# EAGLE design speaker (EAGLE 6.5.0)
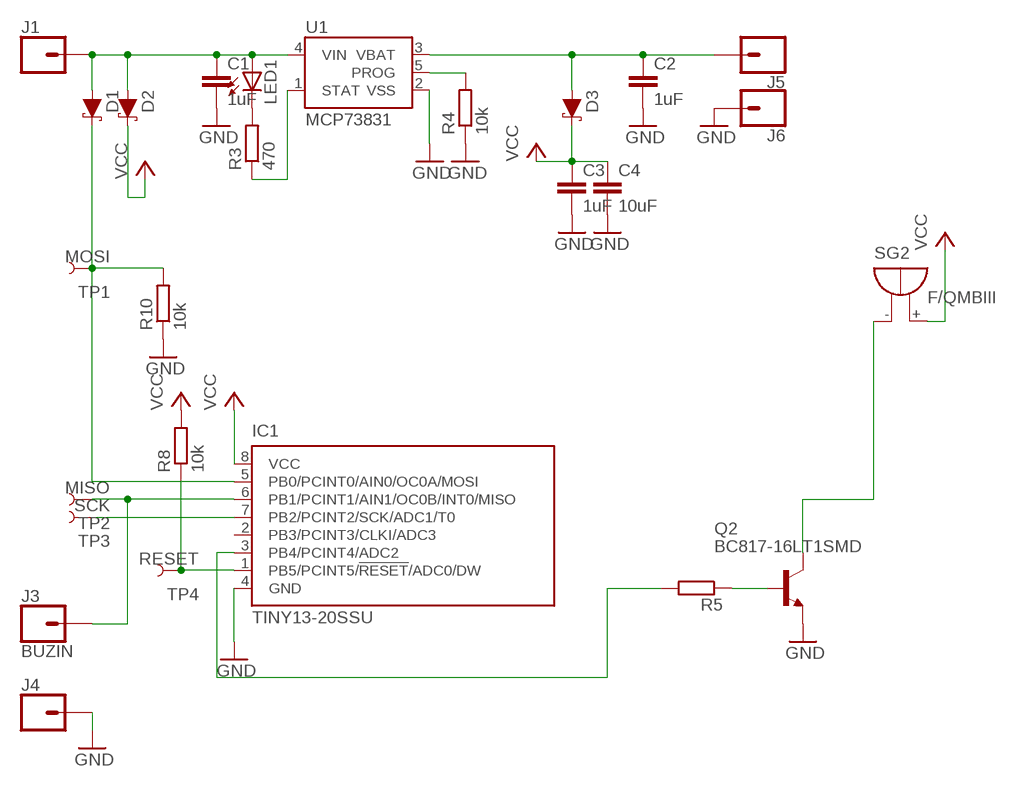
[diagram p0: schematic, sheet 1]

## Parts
C1  1uF  C-EUC1206  [C1206]
C2  1uF  C-EUC1206  [C1206]
C3  1uF  C-EUC1206  [C1206]
C4  10uF  C-EUC1206  [C1206]
D1  DIODE-SCHOTTKY-B340A  [SMA-DIODE]
D2  DIODE-SCHOTTKY-B340A  [SMA-DIODE]
D3  DIODE-SCHOTTKY-B340A  [SMA-DIODE]
IC1  TINY13-20SSU  [8S1]
J1  CONN_01OFFSET  [1X01_OFFSET]
J3  BUZIN  CONN_01OFFSET  [1X01_OFFSET]
J4  CONN_01OFFSET  [1X01_OFFSET]
J5  CONN_01OFFSET  [1X01_OFFSET]
J6  CONN_01OFFSET  [1X01_OFFSET]
LED1  LEDCHIP-LED0805  [CHIP-LED0805]
Q2  BC817-16LT1SMD  [SOT23-BEC]
R3  470  R-EU_M0805  [M0805]
R4  10k  R-EU_M0805  [M0805]
R5  R-EU_M0805  [M0805]
R8  10k  R-EU_M0805  [M0805]
R10  10k  R-EU_M0805  [M0805]
SG2  F/QMBIII  [F/QMBIII]
TP1  MOSI  TEST-POINT3X5  [PAD.03X.05]
TP2  MISO  TEST-POINT3X5  [PAD.03X.05]
TP3  SCK  TEST-POINT3X5  [PAD.03X.05]
TP4  RESET  TEST-POINT3X5  [PAD.03X.05]
U1  MCP73831  [SOT23-5]

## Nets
BUZER: Q2.C SG2.-(+)
GND: C1.2 C2.2 C3.2 C4.2 IC1.4(GND) J4.1 J6.1 Q2.E R4.1 R10.1 U1.2(VSS)
N$3: C1.1 D1.A D2.A J1.1 LED1.A U1.4(VIN)
N$4: LED1.C R3.2
N$6: R3.1 U1.1(STAT)
N$7: R4.2 U1.5(PROG)
N$8: C2.1 D3.A J5.1 U1.3(VBAT)
N$9: IC1.6(PB1/PCINT1/AIN1/OC0B/INT0/MISO) J3.1 TP2.P$1
N$10: IC1.1(PB5/PCINT5/!RESET!/ADC0/DW) R8.1 TP4.P$1
N$12: D1.C IC1.5(PB0/PCINT0/AIN0/OC0A/MOSI) R10.2 TP1.P$1
N$13: IC1.7(PB2/PCINT2/SCK/ADC1/T0) TP3.P$1
N$18: Q2.B R5.1
N$20: IC1.3(PB4/PCINT4/ADC2) R5.2
VCC: C3.1 C4.1 D2.C D3.C IC1.8(VCC) R8.2 SG2.+(-)
Unconnected: IC1.2(PB3/PCINT3/CLKI/ADC3)

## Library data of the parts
C1-C4 = rcl:C-EU: CAPACITOR, European symbol
D1-D3 = SparkFun-DiscreteSemi:DIODE-SCHOTTKY: Schottky diode; PROD_ID: DIO-09886; VALUE: 3A/40V/500mV
IC1 = atmel:TINY13: 8-bit AVR Microcontroller with 1K Bytes In-System Programmable Flash Source: http://www.atmel.com/dyn/resources/prod_documents/2535S.pdf; MPN: ATTINY13-20SSU; OC_FARNELL: 1455133; OC_NEWARK: 58M3771
J1 J3-J6 = SparkFun-Connectors:CONN_01: Single connection point. Often used as Generic Header-pin footprint for 0.1 inch spaced/style header connections
LED1 = led:LED: LED
Q2 = transistor-npn:BC817*: NPN Transistor
R3-R5 R8 R10 = rcl:R-EU_: RESISTOR, European symbol
SG2 = buzzer:F/QMBIII: BUZZER; OC_FARNELL: unknown; OC_NEWARK: unknown
TP1-TP4 = SparkFun-Connectors:TEST-POINT: SparkFun Test Points
U1 = SparkFun-IC-Power:MCP73831: MCP73831T Li-Ion, Li-Pol Controller Miniature single cell, fully integrated Li-Ion, Li-polymer charge management controller Datasheet SparkFun Products: SparkFun ESP32 Thing SparkFun 9DoF Razor IMU M0; PROD_ID: IC-09995

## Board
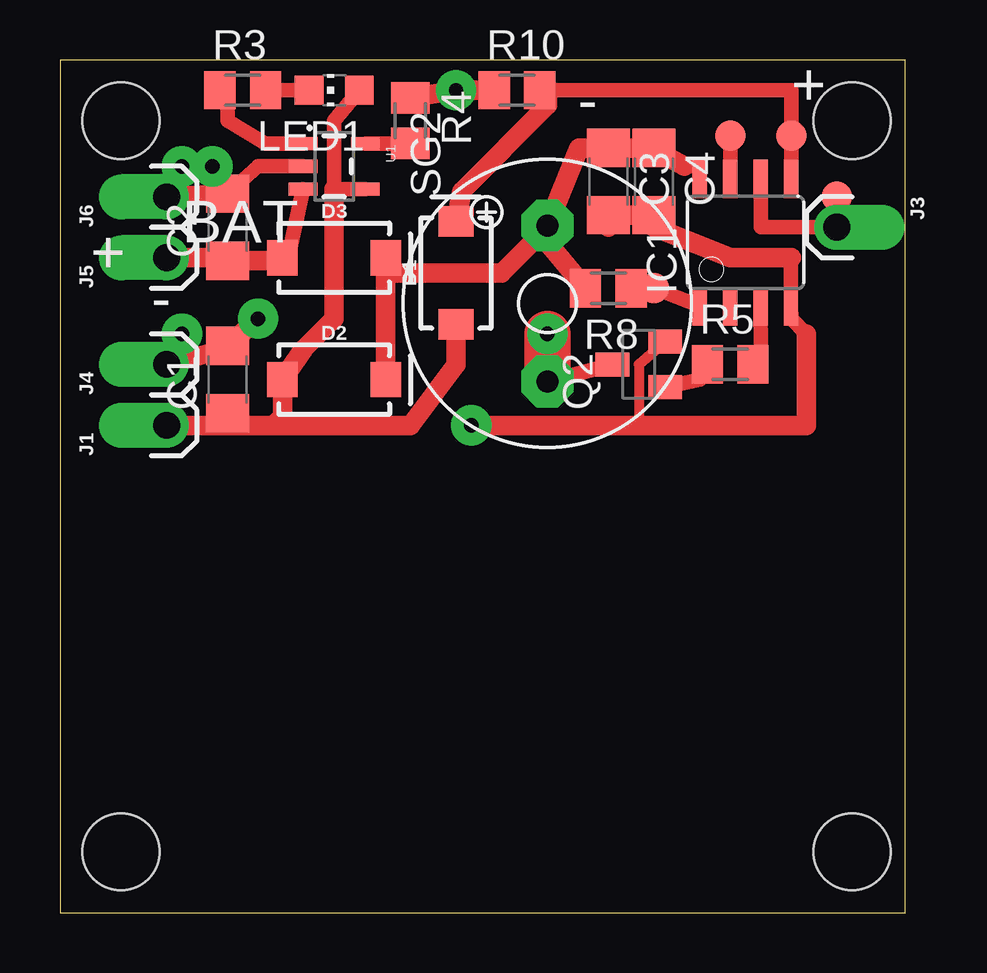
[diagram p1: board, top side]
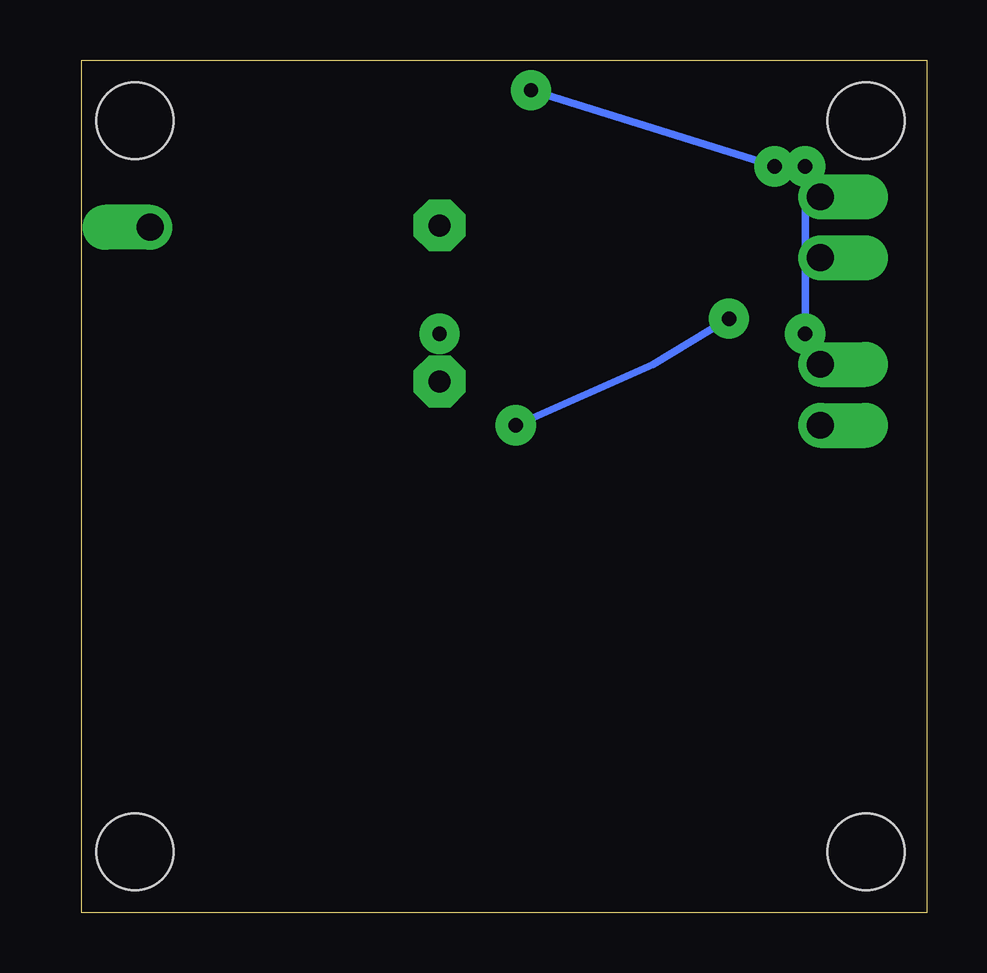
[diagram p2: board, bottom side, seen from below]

Size 35.23 x 35.55 mm. Coordinates in mm from the lower left corner, seen from the top.
Outline: 0,0 35.23,0 35.23,35.55 0,35.55 0,0
Copper layers (1*16): Top 0.035mm / dielectric 1.5mm / Bottom 0.035mm
Design rules "default": minimum track width 10mil, minimum drill 24mil, track to track 8mil, track to pad 8mil, pad to pad 8mil, via to via 8mil, smd to smd 8mil, copper to edge 40mil, drill to drill 8mil, minimum pad ring 10mil, minimum via ring 8mil, stop-mask expansion 4mil, vias tented up to drill 0mil, thermal gap 10mil
Holes 3.2 mm at 2.54,2.54 33.02,2.54 33.02,33.02 2.54,33.02

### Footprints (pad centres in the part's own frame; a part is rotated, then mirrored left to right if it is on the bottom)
C1206 = smd 1.6 x 1.8: 1 -1.4,0; 2 1.4,0
SMA-DIODE = smd 1.27 x 1.47: A -2.15,0; C 2.15,0
8S1 = smd 0.6 x 1.6: 1 -1.905,-2.654; 2 -0.645,-2.654; 3 0.625,-2.654; 4 1.895,-2.654; 5 1.905,2.654; 6 0.635,2.654; 7 -0.635,2.654; 8 -1.905,2.654
1X01_OFFSET = drill 1.118 pad 1.88 offset: 1 0,0
CHIP-LED0805 = smd 1.2 x 1.2: A 0,-1.05; C 0,1.05
SOT23-BEC = smd 1 x 1.4: B -0.95,-1.1; C 0,1.1; E 0.95,-1.1
M0805 = smd 1.3 x 1.6: 1 -0.95,0; 2 0.95,0
F/QMBIII = drill 0.914 pad 2.159 octagon: + 3.251,0; - -3.251,0
PAD.03X.05 = smd 1.27 x 1.27: P$1 0,0
SOT23-5 = smd 0.55 x 1.2: 1 -0.95,-1.3; 2 0,-1.3; 3 0.95,-1.3; 4 0.95,1.3; 5 -0.95,1.3

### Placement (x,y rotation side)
C1  6.99,22.23 90 top
C2  6.99,28.57 90 top
C3  22.86,30.48 270 top
C4  24.77,30.48 270 top
D1  16.51,26.67 90 top
D2  11.43,22.23 0 top
D3  11.43,27.3 0 top
IC1  28.57,27.94 0 top
J1  4.45,20.32 90 top
J3  32.38,28.57 270 top
J4  4.45,22.86 90 top
J5  4.45,27.3 90 top
J6  4.45,29.84 90 top
LED1  11.43,34.29 90 top
Q2  24.13,22.86 90 top
R3  7.62,34.29 0 top
R4  14.61,33.02 270 top
R5  27.94,22.86 0 top
R8  22.86,26.04 180 top
R10  19.05,34.29 0 top
SG2  20.32,25.4 90 top
TP1  30.48,32.38 0 top
TP2  32.38,29.84 0 top
TP3  27.94,32.38 0 top
TP4  24.77,26.04 0 top
U1  11.43,31.11 270 top

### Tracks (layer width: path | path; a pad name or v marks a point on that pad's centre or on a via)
BUZER
  Top 0.61: Q2.C SG2.-
GND  (via drill 0.6 pad 1.68)
  Top 0.406: Q2.E 24.13,22.86 24.13,20.32
  Top 0.61: U1.2 8.26,31.11 C2.2 | 30.48,27.3 30.47,27.3 IC1.4 30.48,24.77 31.11,24.13
  Top 0.813: 30.48,27.3 27.94,27.3 24.77,28.57 C4.2 C3.2 22.86,28.57 | v8.26,24.77 C1.2 6.86,23.5 J4.1 v5.08,24.13 | C2.2 J6.1 v5.08,31.11 v6.35,31.11 | R10.1 v16.51,34.29 R4.1 | 31.11,24.13 31.11,20.32 24.13,20.32 v17.14,20.32
  Bottom 0.305: v17.14,20.32 11.43,22.86 v8.26,24.77 | v5.08,31.11 v5.08,24.13 | v16.51,34.29 v6.35,31.11
N$1  (via drill 0.6 pad 1.68)
  Top 1.93: 20.32,22.23 v20.32,24.13
N$3
  Top 0.61: U1.4 11.43,30.16 11.43,33.02 LED1.A
  Top 0.813: 11.43,30.16 11.43,24.77 10.16,23.5 D2.A 9.28,20.71 8.89,20.32 | D1.A 16.51,22.86 14.61,20.32 8.89,20.32 | J1.1 6.99,20.32 | 6.99,20.32 8.89,20.32 | C1.1 6.99,20.32
N$4
  Top 0.61: R3.2 LED1.C
N$6
  Top 0.61: U1.1 8.57,32.06 6.99,33.02 6.99,34.29 R3.1
N$7
  Top 0.61: U1.5 13.02,32.06 R4.2
N$8
  Top 0.61: U1.3 9.49,27.2 8.26,27.18
  Top 0.813: J5.1 6.22,27.3 C2.1 8.26,27.18 9.15,27.18 D3.A
N$9
  Top 0.61: IC1.6 29.21,28.57 J3.1 TP2.P$1
N$10
  Top 0.61: IC1.1 TP4.P$1 24.13,26.04 R8.1
N$12
  Top 0.61: IC1.5 TP1.P$1 30.48,34.29 R10.2
  Top 0.813: D1.C 16.75,30.09 20.32,33.66 20.32,33.97 R10.2
N$13
  Top 0.61: TP3.P$1 IC1.7
N$18
  Top 0.61: Q2.B 26.67,22.23 R5.1
N$20
  Top 0.61: IC1.3 29.21,23.5 R5.2
VCC
  Top 0.61: IC1.8 26.67,31.11 26.04,31.11
  Top 0.813: 26.04,31.11 24.89,31.75 C4.1 C3.1 21.64,31.88 SG2.+ 20.32,28.57 | D2.C 13.58,26.67 | 13.58,26.67 D3.C | 13.58,26.67 18.41,26.67 20.32,28.57 | R8.2 20.32,27.94 20.32,28.57

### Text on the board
tNames: + | - | BAT | + | -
